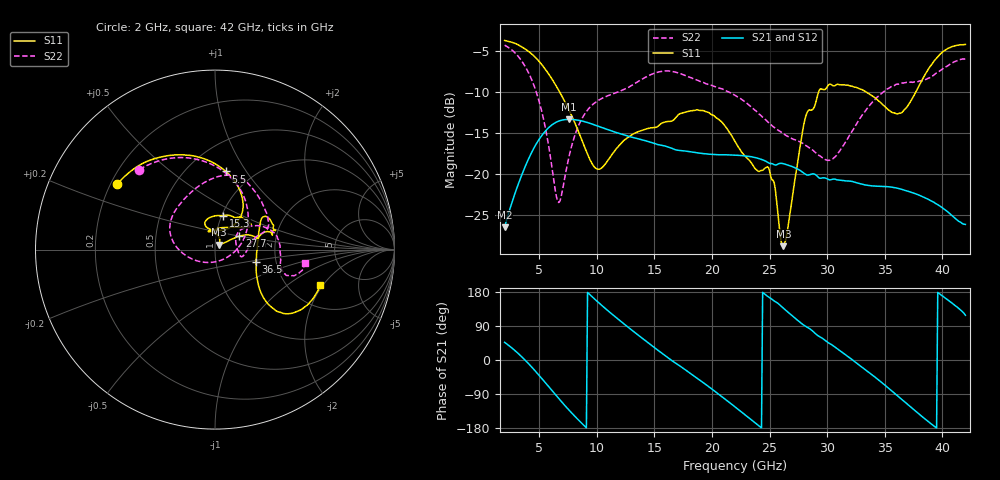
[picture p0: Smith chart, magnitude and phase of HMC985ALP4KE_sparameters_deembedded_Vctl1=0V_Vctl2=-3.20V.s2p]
!s2p File: Measurements: S11, S21, S12, S22
# GHz S dB R 50.0
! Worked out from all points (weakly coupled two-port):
!   401 points, 2 GHz to 42 GHz, reference 50 ohm
!   highest |S21| = -13.34 dB at 7.6 GHz (marker M1); lowest = -26.6 dB at 2 GHz (marker M2)
!   lowest |S11| = -28.9 dB at 26.2 GHz (marker M3), VSWR 1.07, Z = 52.3 + j2.9 ohm
!   |S11| at or under -10 dB: 6.783 GHz to 29.25 GHz (22.47 GHz wide, 125 % of centre); 33.4 GHz to 37.69 GHz (4.292 GHz wide, 12.1 % of centre)
!   |S22| runs from -23.5 to -4.2 dB; largest |S21 - S12| = 0.0007
!   S11 on the Smith chart (normalised r, x): 2 GHz: 0.23, +0.29; 5.5 GHz: 0.75, +0.81; 15.3 GHz: 1.02, +0.40; 27.7 GHz: 1.30, +0.20; 36.5 GHz: 1.57, -0.22; 42 GHz: 2.93, -1.89
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2  -3.67 146.0  -26.56 46.7  -26.55 46.7  -4.25 133.4
3.6  -4.55 118.6  -19.76 5.2  -19.77 5.1  -6.44 92.6
5.5  -7.14 82.1  -14.84 -58.7  -14.85 -58.7  -14.11 28.3
6.6  -9.54 63.4  -13.61 -98.3  -13.61 -98.3  -23.34 -60.2
7.6  -12.23 52.8  -13.34 -132.5  -13.35 -132.5  -17.83 -153.2
8.7  -15.86 53.7  -13.53 -167.1  -13.53 -167.1  -13.28 175.5
10.2  -19.44 88.4  -14.22 150.3  -14.20 150.3  -10.96 152.8
12.5  -15.77 110.0  -15.32 91.9  -15.29 92.0  -9.59 120.3
15.3  -14.20 76.1  -16.43 25.9  -16.44 25.9  -7.56 81.8
15.4  -14.08 74.8  -16.47 23.7  -16.47 23.7  -7.52 80.8
19.2  -12.26 33.6  -17.53 -58.7  -17.52 -58.7  -8.81 41.2
22  -16.02 51.8  -17.72 -123.6  -17.74 -123.7  -10.39 20.4
24.9  -19.23 104.1  -18.67 166.5  -18.63 166.5  -13.71 11.2
26.2  -28.88 50.5  -18.77 136.7  -18.80 136.7  -15.10 -2.8
27.7  -16.24 28.9  -19.65 98.2  -19.65 98.2  -16.16 -14.6
28.7  -12.17 12.9  -20.02 77.4  -20.02 77.4  -17.05 -12.4
30.6  -9.24 19.7  -20.65 35.6  -20.66 35.6  -18.03 22.8
33.2  -9.83 34.3  -21.36 -22.9  -21.34 -22.9  -12.54 33.9
35.4  -12.25 11.8  -21.62 -76.2  -21.60 -76.2  -9.49 17.4
36.5  -12.50 -16.5  -21.93 -104.6  -21.94 -104.6  -8.88 7.8
39.5  -5.84 -43.5  -23.71 -179.4  -23.67 -179.4  -7.65 -19.2
42  -4.15 -18.7  -26.21 118.1  -26.21 118.1  -5.89 -8.3
